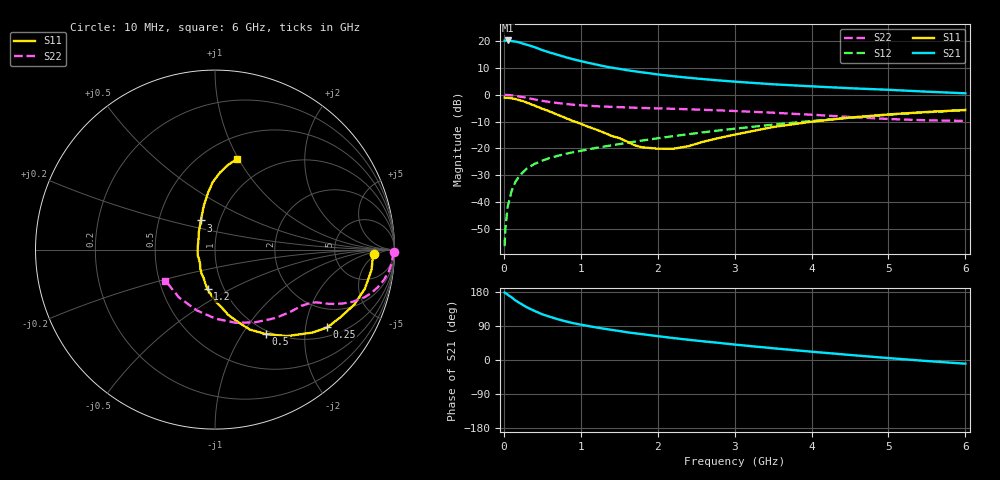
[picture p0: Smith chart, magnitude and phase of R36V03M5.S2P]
! SIEMENS Small Signal Semiconductors
! BFR181
! Si NPN RF Bipolar Junction Transistor in SOT23
! VCE = 6 V  IC = 3.5 mA
! Common Emitter S-Parameters:  May  1996
# GHz  S  MA  R  50
!  f  S11  S21  S12  S22
! GHz  MAG  ANG  MAG  ANG  MAG  ANG  MAG  ANG
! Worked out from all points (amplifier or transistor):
!   36 points, 10 MHz to 6 GHz, reference 50 ohm
!   highest |S21| = 20.3 dB at 50 MHz (marker M1)
!   |S21| within 3 dB of that: start of sweep to 445.6 MHz
!   unconditionally stable (mu >= 1): 1.328 GHz to 3.18 GHz
!   at 250 MHz: K = 0.33, MSG = 24.0 dB, |S12| = -28.8 dB
!   at 1.4 GHz: K = 1.02, MAG = 13.7 dB, |S12| = -18.9 dB
!   at 6 GHz: K = 0.86, MSG = 3.1 dB, |S12| = -5.7 dB
!   S11 on the Smith chart (normalised r, x): 10 MHz: 16, -3; 250 MHz: 1.28, -2.64; 500 MHz: 0.95, -1.28; 1.2 GHz: 0.84, -0.39; 3 GHz: 0.81, +0.27; 6 GHz: 0.71, +0.99
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0.01  0.8854 -1.5  10.25 178.2  0.0015 87.5  0.9949 -0.7
0.02  0.8804 -3.0  10.19 176.6  0.0032 84.6  0.992 -1.4
0.05  0.8792 -7.5  10.32 172.4  0.0082 87.3  0.9896 -3.6
0.15  0.8332 -21.7  9.833 157.4  0.0236 77.8  0.9561 -10.2
0.2  0.7936 -28.4  9.505 151.0  0.0305 74.5  0.9299 -13.1
0.25  0.7611 -34.7  8.99 144.9  0.0361 71.1  0.904 -15.5
0.3  0.7144 -40.3  8.56 139.0  0.0423 69.2  0.8758 -17.6
0.4  0.6272 -50.2  7.737 129.4  0.0515 65.4  0.8196 -20.8
0.5  0.5496 -58.9  6.821 120.6  0.0592 63.1  0.7697 -23.0
0.6  0.4867 -66.4  6.132 113.9  0.0666 61.5  0.733 -24.4
0.7  0.4233 -72.4  5.565 107.7  0.0726 60.5  0.7011 -25.5
0.8  0.3705 -78.6  5.041 102.1  0.0791 59.9  0.6765 -26.3
0.9  0.3232 -83.6  4.607 97.3  0.0846 59.9  0.6533 -26.9
1.1  0.2521 -94.9  3.945 89.6  0.096 60.2  0.6229 -28.3
1.2  0.2246 -100.7  3.668 85.9  0.1021 60.5  0.6128 -29.0
1.6  0.1345 -127.6  2.878 73.2  0.127 60.6  0.582 -32.2
2.2  0.0983 165.6  2.222 58.0  0.1692 60.4  0.5473 -38.8
3  0.1806 115.9  1.759 40.7  0.2329 57.0  0.4988 -50.7
3.5  0.2507 104.5  1.571 31.0  0.2774 53.6  0.4633 -60.9
4.5  0.3755 92.0  1.326 13.3  0.3747 44.2  0.3853 -89.3
5.5  0.4781 81.2  1.143 -2.7  0.4723 31.9  0.3337 -126.9
6  0.5209 76.2  1.066 -9.8  0.5178 24.9  0.3263 -147.9
